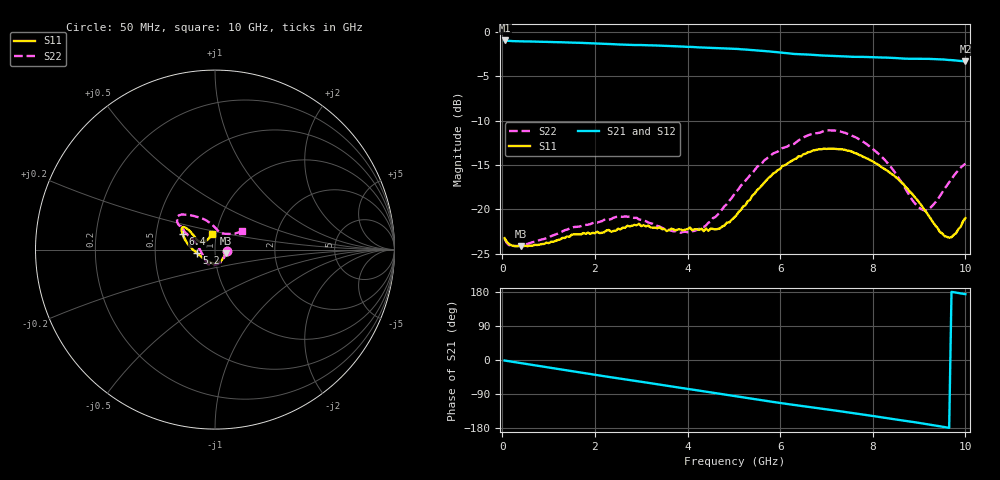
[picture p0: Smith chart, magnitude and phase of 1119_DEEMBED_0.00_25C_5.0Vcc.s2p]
!Hittite Microwave Corp.
!Digital Attenuator/PhaseShifter Rev 1.4.0
!Filename: C:\DATA\DATA\1119_DEEMBED_0.00_25C_5.0Vcc.s2p
!VNA ID: Agilent Technologies,N5224A,MY51441122,A.10.45.03
!Device type:
!2 Port Calibration.
!Temp(C): 25
!Lot Number:
!Serial Number:
!Operator:
!Misc:
!Attenuator:  0.000
# GHZ S DB R 50.0
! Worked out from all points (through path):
!   200 points, 50 MHz to 10 GHz, reference 50 ohm
!   highest |S21| = -0.99 dB at 50 MHz (marker M1); lowest = -3.4 dB at 10 GHz (marker M2)
!   group delay of S21, straight-line fit = 50.9 ps
!   lowest |S11| = -24.1 dB at 400 MHz (marker M3), VSWR 1.13, Z = 56.2 - j2.21 ohm
!   |S11| at or under -10 dB: start of sweep to end of sweep
!   |S22| runs from -24.1 to -11.1 dB; largest |S21 - S12| = 0.0022
!   S11 on the Smith chart (normalised r, x): 50 MHz: 1.15, -0.02; 5.2 GHz: 0.81, -0.03; 6.4 GHz: 0.69, +0.12; 10 GHz: 0.96, +0.17
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0.05  -23.24 -7.0  -0.99 -1.4  -0.98 -1.4  -23.32 -7.4
0.15  -23.92 -10.0  -1.04 -3.3  -1.04 -3.3  -24.03 -10.9
0.4  -24.14 -18.4  -1.09 -8.1  -1.08 -8.1  -24.05 -20.6
1.75  -22.66 -71.3  -1.26 -34.1  -1.26 -34.1  -21.79 -75.7
2.65  -22.07 -85.4  -1.48 -51.0  -1.47 -51.1  -20.78 -108.2
3.4  -22.01 -99.0  -1.57 -64.9  -1.56 -65.0  -21.95 -134.5
3.85  -22.26 -105.5  -1.67 -73.4  -1.67 -73.5  -22.63 -149.3
4.35  -22.45 -119.3  -1.79 -82.6  -1.80 -82.7  -21.98 -174.8
4.7  -22.14 -138.1  -1.87 -89.1  -1.88 -89.2  -20.31 168.7
5.05  -20.71 -160.3  -1.94 -95.7  -1.96 -95.7  -18.05 157.6
5.2  -19.68 -170.1  -1.99 -98.5  -2.00 -98.6  -17.06 154.8
5.85  -15.96 166.9  -2.27 -110.7  -2.28 -110.8  -13.70 148.2
6.4  -14.01 154.5  -2.54 -120.0  -2.55 -120.1  -12.23 145.8
6.7  -13.39 150.2  -2.61 -125.2  -2.62 -125.2  -11.50 142.7
7.45  -13.38 144.3  -2.80 -137.9  -2.81 -138.0  -11.48 132.9
7.9  -14.32 143.2  -2.85 -145.9  -2.87 -146.0  -12.78 124.2
8.35  -15.79 144.5  -2.93 -154.2  -2.94 -154.2  -14.97 109.4
8.9  -18.58 150.8  -3.05 -164.0  -3.05 -164.1  -19.27 82.8
9.1  -19.94 152.7  -3.06 -167.9  -3.07 -167.9  -20.10 69.8
9.3  -21.44 151.6  -3.07 -171.9  -3.09 -171.9  -19.52 56.4
9.65  -23.18 129.8  -3.19 -179.1  -3.20 -179.1  -16.96 39.0
10  -20.97 99.4  -3.35 173.7  -3.36 173.7  -14.86 34.7
